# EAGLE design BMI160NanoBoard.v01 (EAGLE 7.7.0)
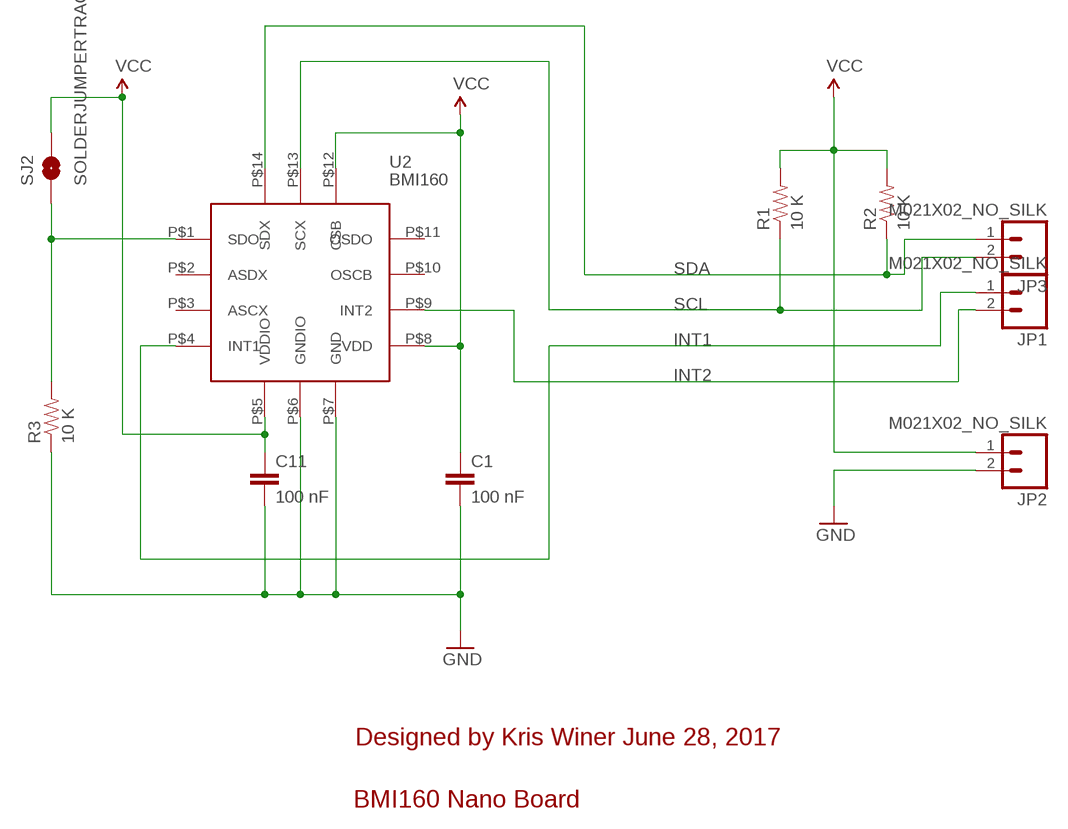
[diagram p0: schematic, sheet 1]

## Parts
C1  100 nF  0402CAP.KW  [0402-CAP]
C11  100 nF  0402CAP.KW  [0402-CAP]
JP1  M021X02_NO_SILK  [1X02_NO_SILK]
JP2  M021X02_NO_SILK  [1X02_NO_SILK]
JP3  M021X02_NO_SILK  [1X02_NO_SILK]
R1  10 K  0402RES.KW  [0402-RES]
R2  10 K  0402RES.KW  [0402-RES]
R3  10 K  0402RES.KW  [0402-RES]
SJ2  SOLDERJUMPERTRACE  [SJ_2S-TRACE]
U2  BMI160  [BMI160]

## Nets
GND: C1.2 C11.2 JP2.2 R3.1 U2.P$6(GNDIO) U2.P$7(GND)
INT1: JP1.1 U2.P$4(INT1)
INT2: JP1.2 U2.P$9(INT2)
N$2: R3.2 SJ2.1 U2.P$1(SDO)
SCL: JP3.2 R1.1 U2.P$13(SCX)
SDA: JP3.1 R2.1 U2.P$14(SDX)
VCC: C1.1 C11.1 JP2.1 R1.2 R2.2 SJ2.2 U2.P$5(VDDIO) U2.P$8(VDD) U2.P$12(CSB)
Unconnected: U2.P$2(ASDX) U2.P$3(ASCX) U2.P$10(OSCB) U2.P$11(OSDO)

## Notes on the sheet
- Designed by Kris Winer June 28, 2017
- BMI160 Nano Board

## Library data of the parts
C1 C11 = SparkFun-Capacitors:0402CAP.KW
JP1-JP3 = SparkFun-Connectors:M02: Standard 2-pin 0.1" header. Use with
R1-R3 = SparkFun-Resistors:0402RES.KW
SJ2 = SparkFun-Passives:SOLDERJUMPER: Solder Jumper
U2 = kris:BMI160: Bosch BMI160 accel/gyro

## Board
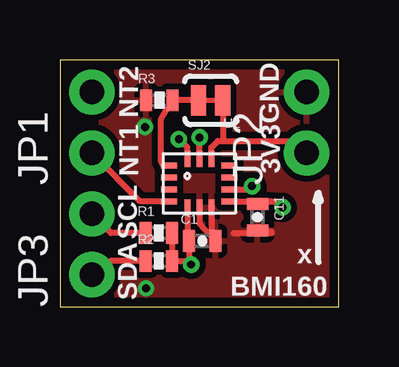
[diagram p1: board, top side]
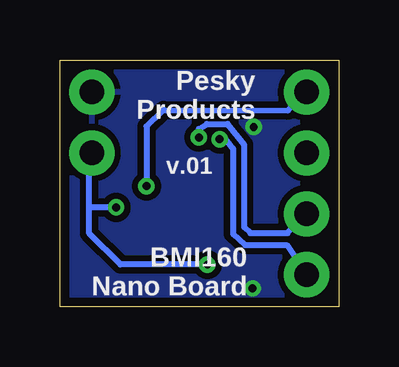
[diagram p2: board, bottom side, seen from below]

Size 11.63 x 10.29 mm. Coordinates in mm from the lower left corner, seen from the top.
Outline: 0,0 11.63,0 11.63,10.29 0,10.29 0,0
Copper layers (1*16): Top 0.0356mm / dielectric 1.5011mm / Bottom 0.0356mm
Design rules "OSHPark *": minimum track width 6mil, minimum drill 13mil, track to track 6mil, track to pad 6mil, pad to pad 6mil, via to via 6mil, smd to smd 6mil, copper to edge 15mil, drill to drill 6mil, minimum pad ring 7mil, minimum via ring 7mil, stop-mask expansion 3mil, vias tented up to drill 20mil, thermal gap 10mil

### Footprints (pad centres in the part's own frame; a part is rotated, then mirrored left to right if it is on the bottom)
0402-CAP = smd 0.5 x 0.9: 1 -0.55,0; 2 0.55,0
1X02_NO_SILK = drill 1.016 pad 1.88: 1 0,0; 2 2.54,0
0402-RES = smd 0.5 x 0.9: 1 -0.55,0; 2 0.55,0
SJ_2S-TRACE = smd 0.635 x 1.27: 1 -0.508,0; 2 0.508,0
BMI160 = smd 0.675 x 0.25: P$1 -1.262,0.75; P$2 -1.262,0.25; P$3 -1.262,-0.25; P$4 -1.262,-0.75; P$8 1.262,-0.75; P$9 1.262,-0.25; P$10 1.262,0.25; P$11 1.262,0.75 | smd 0.25 x 0.675: P$5 -0.5,-1.012; P$6 0,-1.012; P$7 0.5,-1.012; P$12 0.5,1.012; P$13 0,1.012; P$14 -0.5,1.012

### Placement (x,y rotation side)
C1  5.93,2.74 0 top
C11  8.24,3.73 270 top
JP1  1.33,6.41 90 top
JP2  10.29,6.41 90 top
JP3  1.33,1.33 90 top
R1  4.13,3.07 0 top
R2  4.13,1.9 0 top
R3  4.15,8.61 0 top
SJ2  6.29,8.61 0 top
U2  5.81,5.15 0 top

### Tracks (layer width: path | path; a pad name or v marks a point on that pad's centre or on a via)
GND  (via drill 0.33)
  Top 0.254: 7.25,3.07 8.84,3.07 8.84,3.12 C11.2 | U2.P$7 6.32,2.94 C1.2 5.82,3.48 U2.P$6
  other vias: 3.54,7.49 3.59,0.76
  pour Top (isolate 0.254): 0,10.29 11.62,10.29 11.62,0 0,0
  pour Bottom (isolate 0.254): 0,10.29 11.62,10.29 11.62,0 0,0
INT1
  Top 0.254: U2.P$4 3.35,4.4 JP1.1
INT2  (via drill 0.33)
  Top 0.254: U2.P$9 7.78,4.9 v8.01,5.03
  Bottom 0.254: JP1.2 2.11,8.18 7.3,8.2 8.01,7.52 v8.01,5.03
N$2
  Top 0.254: SJ2.1 R3.2 4.23,7.83 4.23,6.02 4.31,5.9 U2.P$1
SCL  (via drill 0.33)
  Top 0.254: R1.1 2.13,3.07 JP3.2 | U2.P$13 5.82,6.75 v5.83,7.06
  Bottom 0.254: v5.83,7.06 5.83,7.42 5.5,7.62 4.64,7.62 3.95,6.76 3.95,3.32 3.68,3.07 2.13,3.07 JP3.2
SDA  (via drill 0.33)
  Top 0.254: R2.1 2.11,1.9 JP3.1 | U2.P$14 5.31,6.64 v4.97,6.98
  Bottom 0.254: v4.97,6.98 4.71,6.98 4.41,6.58 4.41,3.02 3.9,2.57 2.16,2.57 JP3.1
VCC  (via drill 0.33)
  Top 0.254: U2.P$5 5.32,3.07 C1.1 5.38,1.96 v5.47,1.75 5.32,1.9 R2.2 R1.2 | U2.P$8 8.79,4.4 | 8.79,4.4 C11.1 | U2.P$12 6.32,6.61 6.32,6.64 6.59,6.91 6.77,6.91 | 6.77,6.91 9.68,6.91 JP2.1 | 8.79,4.4 8.96,4.4 v9.28,4.14 | SJ2.2 6.79,6.93 6.77,6.91
  Bottom 0.254: v5.47,1.75 9.11,1.75 10.4,3.05 10.4,4.11 | v9.28,4.14 10.35,4.14 10.4,4.11 | 10.4,4.11 10.4,6.31 JP2.1

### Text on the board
tPlace: NT2 | GND | NT1 | 3V3 | SCL | x | BMI160 | SDA
bPlace: Pesky / Products | v.01 | BMI160 / Nano Board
